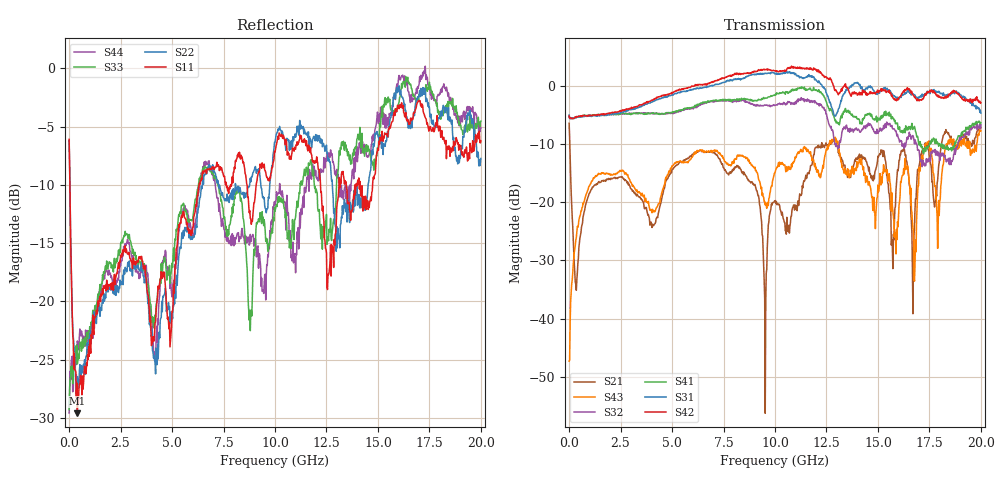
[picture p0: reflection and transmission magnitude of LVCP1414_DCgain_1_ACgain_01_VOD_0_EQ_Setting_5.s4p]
!Agilent Technologies,N5230A,MY46400459,A.07.50.48
!Agilent N5230A: A.07.50.48
!Date: Tuesday, April 17, 2012 18:46:38
!Correction: S11(Full 4 Port(1,2,3,4))
!S12(Full 4 Port(1,2,3,4))
!S13(Full 4 Port(1,2,3,4))
!S14(Full 4 Port(1,2,3,4))
!S21(Full 4 Port(1,2,3,4))
!S22(Full 4 Port(1,2,3,4))
!S23(Full 4 Port(1,2,3,4))
!S24(Full 4 Port(1,2,3,4))
!S31(Full 4 Port(1,2,3,4))
!S32(Full 4 Port(1,2,3,4))
!S33(Full 4 Port(1,2,3,4))
!S34(Full 4 Port(1,2,3,4))
!S41(Full 4 Port(1,2,3,4))
!S42(Full 4 Port(1,2,3,4))
!S43(Full 4 Port(1,2,3,4))
!S44(Full 4 Port(1,2,3,4))
!S4P File: Measurements: <S11,S12,S13,S14>,
!<S21,S22,S23,S24>,
!<S31,S32,S33,S34>,
!<S41,S42,S43,S44>:
# Hz S  dB  R 50
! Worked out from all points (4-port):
!   801 points, 300 kHz to 20 GHz, reference 50 ohm
!   strongest paths, dB at 300 kHz, 5 GHz, 10 GHz, 15 GHz, 20 GHz:
!     S42: -5.2, -1.2, 2.5, -0.9, -2.9
!     S31: -5.1, -1.6, 2.0, -1.3, -4.7
!     S41: -5.1, -4.5, -1.7, -5.6, -6.4
!     S32: -5.2, -4.8, -3.4, -8.2, -6.7
!     S43: -47.3, -13.8, -15.0, -17.1, -7.8
!     S21: -6.5, -14.4, -19.9, -12.1, -7.2
!   lowest |S11| = -29.6 dB at 400.3 MHz (marker M1), VSWR 1.07, Z = 53.1 + j1.44 ohm
!   |S11| at or under -10 dB: 37.35 MHz to 6.31 GHz (6.273 GHz wide, 198 % of centre); 12.21 GHz to 13.11 GHz (897.7 MHz wide, 7.09 % of centre); 14.13 GHz to 14.74 GHz (608.2 MHz wide, 4.21 % of centre)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
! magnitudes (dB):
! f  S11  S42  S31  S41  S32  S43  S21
! 300 kHz  -6.1  -5.2  -5.1  -5.1  -5.2  -47.3  -6.5
! 400.3 MHz  -29.6  -5.4  -5.4  -5.4  -5.4  -24.2  -32.1
! 10.15 GHz  -5.8  2.4  2.1  -1.4  -3.1  -13.6  -20.3
! 12.73 GHz  -17.8  1.1  -3.5  -4.2  -7.0  -9.7  -9.7
! 14.05 GHz  -10.0  -1.4  0.4  -5.7  -7.5  -13.3  -12.1
! 16.8 GHz  -3.7  -1.9  -1.6  -7.4  -9.3  -30.8  -21.2
! 20 GHz  -6.2  -2.9  -4.7  -6.4  -6.7  -7.8  -7.2
